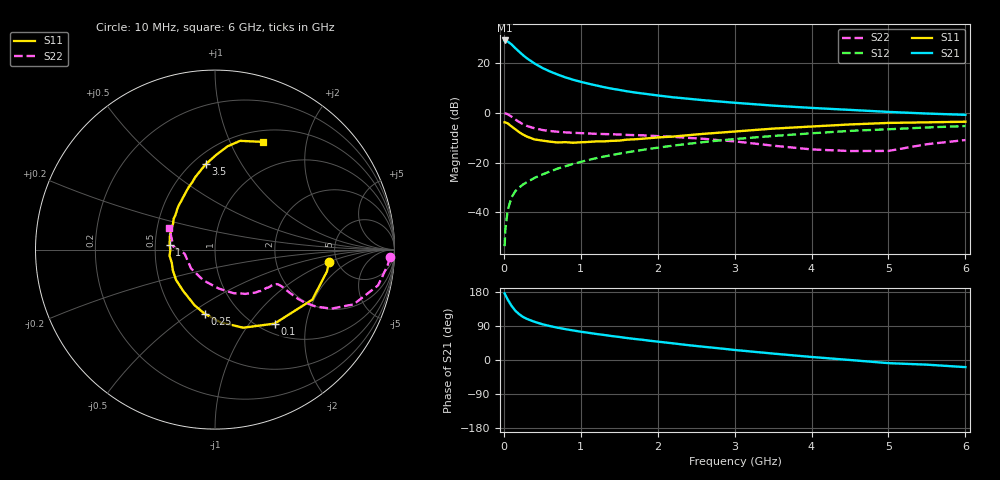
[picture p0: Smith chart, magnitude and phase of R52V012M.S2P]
! SIEMENS Small Signal Semiconductors
! BFR183
! Si NPN RF Bipolar Junction Transistor in SOT23
! VCE = 2 V  IC = 12 mA
! Common Emitter S-Parameters:  May  1996
# GHz  S  MA  R  50
!  f  S11  S21  S12  S22
! GHz  MAG  ANG  MAG  ANG  MAG  ANG  MAG  ANG
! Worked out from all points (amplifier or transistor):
!   36 points, 10 MHz to 6 GHz, reference 50 ohm
!   highest |S21| = 28.9 dB at 10 MHz (marker M1)
!   |S21| within 3 dB of that: start of sweep to 146.2 MHz
!   unconditionally stable (mu >= 1): 682 MHz to 2.462 GHz
!   at 250 MHz: K = 0.69, MSG = 25.9 dB, |S12| = -28.8 dB
!   at 1.4 GHz: K = 1.05, MAG = 11.9 dB, |S12| = -17.0 dB
!   at 6 GHz: K = 0.90, MSG = 2.2 dB, |S12| = -5.4 dB
!   S11 on the Smith chart (normalised r, x): 10 MHz: 4.31, -0.97; 100 MHz: 1.17, -1.34; 250 MHz: 0.70, -0.57; 1 GHz: 0.60, +0.04; 3.5 GHz: 0.58, +0.71; 6 GHz: 0.63, +1.34
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0.01  0.6391 -6.0  28.01 175.8  0.0021 92.6  0.9751 -2.5
0.02  0.6357 -11.0  27.77 171.4  0.0046 83.2  0.966 -5.2
0.05  0.6099 -27.2  26.66 159.7  0.0111 76.8  0.93 -12.4
0.1  0.5292 -51.2  23.33 142.9  0.02 70.8  0.8298 -21.6
0.15  0.4628 -70.1  19.57 129.9  0.0267 65.8  0.727 -26.9
0.2  0.4062 -85.7  16.61 120.7  0.0315 63.9  0.6477 -29.4
0.25  0.362 -99.2  14.18 113.6  0.0363 63.6  0.5841 -30.5
0.3  0.3306 -110.1  12.3 108.4  0.0404 63.8  0.5408 -30.7
0.4  0.29 -128.0  9.666 100.8  0.0492 64.9  0.4849 -30.1
0.5  0.2749 -142.3  7.888 94.4  0.0574 65.5  0.4489 -29.4
0.6  0.2619 -153.6  6.69 89.5  0.0661 66.4  0.4281 -28.9
0.7  0.2519 -162.9  5.802 85.2  0.0755 67.2  0.4136 -28.8
0.8  0.2557 -172.3  5.097 81.4  0.0841 66.6  0.4022 -28.9
1  0.2546 173.7  4.146 74.7  0.1029 66.8  0.3886 -29.8
1.1  0.2583 167.1  3.806 71.8  0.1125 66.4  0.382 -31.0
1.3  0.2652 156.9  3.248 66.1  0.1316 65.3  0.3721 -32.8
1.6  0.2873 143.3  2.68 58.0  0.1597 63.2  0.3573 -36.8
2.2  0.3315 124.2  2.031 43.9  0.2176 57.7  0.3279 -47.1
3.5  0.4778 96.3  1.382 16.9  0.3402 42.0  0.2176 -84.7
4.5  0.5795 83.1  1.135 0.0  0.4307 29.4  0.1698 -141.7
5.5  0.6388 70.6  0.959 -12.3  0.5044 17.4  0.2327 175.8
6  0.6579 65.9  0.903 -18.8  0.5386 9.6  0.2823 154.4
